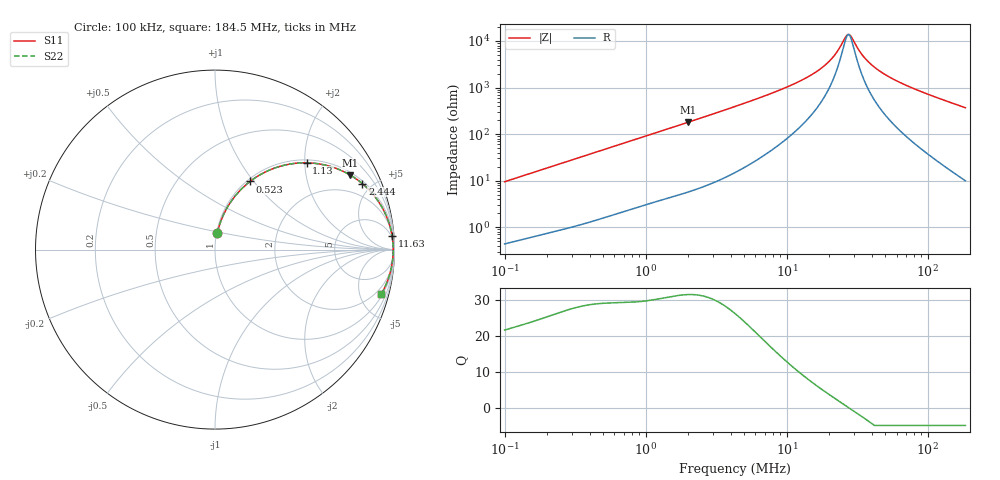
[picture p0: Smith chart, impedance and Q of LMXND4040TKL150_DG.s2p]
! LMXND4040TKL150_DG  S-PARAMETER MODEL  ( General Type )
! Model Generated by TAIYO YUDEN Corporation (https://www.yuden.co.jp/en/)
! Version 1.0
! TAIYO YUDEN Control No. 191023NI43SB-FBB
! Copyright(c) 2019 TAIYO YUDEN CO.,LTD. All Rights Reserved.
! Product Description (link to TY-COMPAS)
! https://ds.yuden.co.jp/TYCOMPAS/or/detail?pn=LMXND4040TKL150MDG&u=M
! Products Name : Inductors
! Characteristics :
!  Inductance : 15 uH , SRF(min) : 18 MHz , DC Resistance(max) : 0.252 Ohm
!  Rated Current : Saturation :1100 mA , Temp Rise : 850 mA (40 degC)
!  Case Size : 4.0 x 4.0 / 0.157 x 0.157 [mm/inch] , Thickness : 1.8 / 0.071 [mm/inch]
!  (Conditions: Temperature = 25 degC , DC Bias Current/Voltage = 0A / 0V)
! External Node Assignments :
!  1  o---GGG---o  2
! GND o---------o GND
! Frequency Range : 0.1MHz  -  184.468258MHz  [ 402 STEP ]
# MHz S RI R 50
! Freq[MHz].  S11 Real  S11 Imag  S21 Real  S21 Imag  S12 Real  S12 Imag  S22 Real  S22 Imag
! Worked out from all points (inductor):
!   401 points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, 100 kHz to 184.5 MHz, reference 50 ohm
!   read as one part in series: L = 15 uH near 103.8 kHz
!   highest Q = 31.6 at 1.987 MHz (marker M1), where L = 14.3 uH
!   self-resonance near 27.11 MHz
!   S11 on the Smith chart (normalised r, x): 100 kHz: 1.01, +0.19; 523 kHz: 1.03, +0.96; 1.13 MHz: 1.07, +2.04; 2.444 MHz: 1.14, +4.39; 11.63 MHz: 3, +25; 184.5 MHz: 1.20, -7.38
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0.1  0.0131 0.0931  0.9869 -0.0931  0.9869 -0.0931  0.0131 0.0931
0.352405  0.1041 0.2882  0.8959 -0.2882  0.8959 -0.2882  0.1041 0.2882
0.523001  0.1953 0.3797  0.8047 -0.3797  0.8047 -0.3797  0.1953 0.3797
0.805922  0.3544 0.4616  0.6456 -0.4616  0.6456 -0.4616  0.3544 0.4616
1.130472  0.5106 0.4835  0.4894 -0.4835  0.4894 -0.4835  0.5106 0.4835
1.241892  0.5552 0.4808  0.4448 -0.4808  0.4448 -0.4808  0.5552 0.4808
1.987027  0.7546 0.4148  0.2454 -0.4148  0.2454 -0.4148  0.7546 0.4148
2.443525  0.8208 0.3679  0.1792 -0.3679  0.1792 -0.3679  0.8208 0.3679
4.294977  0.9309 0.2353  0.0691 -0.2353  0.0691 -0.2353  0.9309 0.2353
11.6331  0.9864 0.0776  0.0136 -0.0776  0.0136 -0.0776  0.9864 0.0776
15.13571  0.9901 0.0508  0.0099 -0.0508  0.0099 -0.0508  0.9901 0.0508
20.44747  0.9922 0.024  0.00778 -0.024  0.00778 -0.024  0.9922 0.024
22.88908  0.9926 0.0146  0.0074 -0.0146  0.0074 -0.0146  0.9926 0.0146
26.10851  0.9928 0.00386  0.00717 -0.00386  0.00717 -0.00386  0.9928 0.00386
27.62336  0.9928 -0.000715  0.00715 0.000715  0.00715 0.000715  0.9928 -0.000715
28.68178  0.9928 -0.00376  0.00716 0.00376  0.00716 0.00376  0.9928 -0.00376
33.33684  0.9926 -0.0161  0.00739 0.0161  0.00739 0.0161  0.9926 -0.0161
37.31757  0.9922 -0.0255  0.00778 0.0255  0.00778 0.0255  0.9922 -0.0255
43.37423  0.9914 -0.0386  0.00862 0.0386  0.00862 0.0386  0.9914 -0.0386
53.33896  0.9895 -0.058  0.0105 0.058  0.0105 0.058  0.9895 -0.058
88.61236  0.9789 -0.117  0.0211 0.117  0.0211 0.117  0.9789 -0.117
184.4683  0.9258 -0.249  0.0742 0.249  0.0742 0.249  0.9258 -0.249
